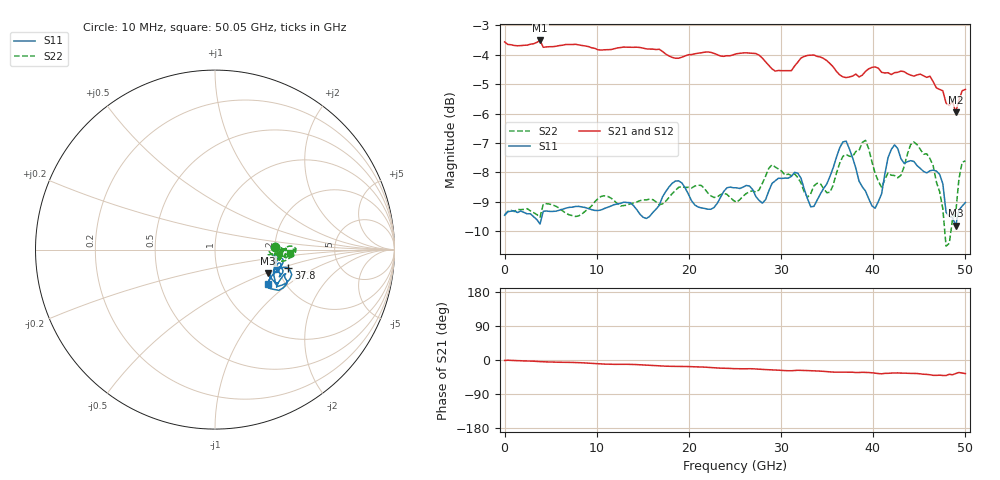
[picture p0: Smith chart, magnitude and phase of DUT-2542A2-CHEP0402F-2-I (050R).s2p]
! Touchstone file from project
! Exported from ElectronicsDesktop 2025.1.3
# GHz S MA R 50.000000
! Terminal data exported
! Port[1] = Port1
! Port[2] = Port2
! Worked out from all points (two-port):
!   144 points, 10 MHz to 50.05 GHz, reference 50 ohm
!   highest |S21| = -3.52 dB at 3.859 GHz (marker M1); lowest = -6.0 dB at 49 GHz (marker M2)
!   |S21| within 3 dB of the highest: start of sweep to end of sweep
!   lowest |S11| = -9.8 dB at 49 GHz (marker M3), VSWR 1.96, Z = 87.4 - j25.4 ohm
!   |S11| at or under -10 dB: nowhere
!   |S22| runs from -10.5 to -6.9 dB; largest |S21 - S12| = 0.011
!   S11 on the Smith chart (normalised r, x): 10 MHz: 2.01, +0.07; 37.8 GHz: 2.29, -0.56; 50.05 GHz: 1.64, -0.73
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0.01  0.3369 2.6  0.6627 -1.3  0.6635 -1.4  0.3374 2.7
! Gamma 0 0 0 0
! Port Impedance 50 0 50 0
3.85945  0.3255 -6.5  0.6666 -4.3  0.6652 -4.3  0.3341 -4.5
8.4088  0.3479 -4.0  0.6536 -7.3  0.6522 -7.2  0.3386 1.1
10.85845  0.3459 -11.7  0.6428 -10.8  0.6412 -10.6  0.3634 -9.0
14.008  0.3498 -4.5  0.649 -11.7  0.6479 -11.5  0.3534 3.3
16.8076  0.3501 -16.4  0.6441 -15.8  0.6424 -15.4  0.3509 -6.2
19.95715  0.3661 -7.4  0.6305 -17.3  0.6303 -17.3  0.3756 -2.0
25.2064  0.375 -18.6  0.6329 -23.0  0.6331 -22.7  0.3544 -8.1
27.3061  0.3622 -11.8  0.6334 -23.7  0.6337 -23.5  0.3686 -1.7
29.05585  0.3815 -19.9  0.5965 -26.1  0.5972 -25.7  0.4102 -4.4
33.6052  0.3488 -20.9  0.6299 -28.5  0.6312 -28.1  0.3778 -5.7
35.7049  0.4059 -30.3  0.6011 -32.0  0.5997 -31.7  0.3795 -10.0
37.8046  0.4216 -13.9  0.58 -32.3  0.5784 -31.9  0.4235 -3.1
39.2044  0.3703 -17.2  0.5908 -32.8  0.5877 -32.5  0.4513 0.6
40.25425  0.3462 -29.0  0.6012 -34.8  0.5995 -34.1  0.3965 1.9
42.004  0.4355 -29.3  0.5835 -34.5  0.584 -34.2  0.3939 1.1
43.4038  0.4125 -20.0  0.5901 -34.7  0.5892 -34.4  0.4075 -6.8
44.45365  0.4157 -18.9  0.58 -35.4  0.5788 -35.0  0.4485 -1.6
46.55335  0.4018 -31.4  0.5675 -40.4  0.5661 -39.5  0.4088 -2.6
47.95315  0.3409 -26.4  0.5221 -41.0  0.5218 -40.1  0.2985 -5.5
49.003  0.3234 -23.7  0.5036 -35.7  0.5018 -34.9  0.3398 -1.1
50.05285  0.3541 -33.0  0.5507 -35.8  0.5502 -34.8  0.4165 -2.6
